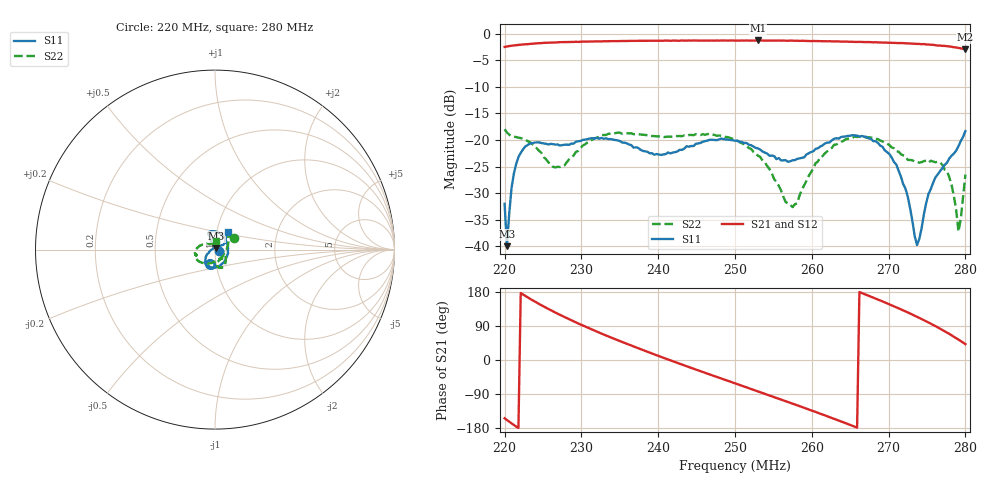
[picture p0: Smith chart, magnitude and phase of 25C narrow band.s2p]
!Agilent Technologies,E8362C,SG49020144,A.09.33.09
!Agilent E8362C: A.09.33.09
!Date: Friday, October 10, 2025 09:41:16
!Correction: S11(Full 2 Port(1,2))
!S21(Full 2 Port(1,2))
!S12(Full 2 Port(1,2))
!S22(Full 2 Port(1,2))
!S2P File: Measurements: S11, S21, S12, S22:
# Hz S  dB  R 50
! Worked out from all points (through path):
!   201 points, 220 MHz to 280 MHz, reference 50 ohm
!   highest |S21| = -1.26 dB at 253 MHz (marker M1); lowest = -2.9 dB at 280 MHz (marker M2)
!   lowest |S11| = -40.0 dB at 220.3 MHz (marker M3), VSWR 1.02, Z = 50.8 + j0.655 ohm
!   |S11| at or under -10 dB: start of sweep to end of sweep
!   |S22| runs from -37.2 to -18.0 dB; largest |S21 - S12| = 0.0071
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2.2e8  -32.01 -15.6  -2.48 -153.7  -2.50 -153.7  -17.98 32.0
2.203e8  -40.00 40.1  -2.39 -158.3  -2.40 -158.2  -18.59 36.2
2.212e8  -26.37 116.5  -2.20 -171.4  -2.19 -171.3  -19.40 44.6
2.224e8  -21.77 111.1  -2.02 172.8  -2.03 172.6  -19.82 45.1
2.266e8  -20.87 107.7  -1.64 125.3  -1.65 125.5  -25.16 -32.7
2.302e8  -19.97 111.6  -1.48 90.9  -1.48 90.8  -21.03 -118.9
2.344e8  -20.00 85.4  -1.38 54.7  -1.38 54.8  -18.72 -152.7
2.401e8  -22.73 5.7  -1.30 10.2  -1.31 10.4  -19.32 -163.6
2.446e8  -21.14 -66.2  -1.26 -23.0  -1.28 -22.8  -19.09 -164.6
2.5e8  -20.12 -111.2  -1.29 -61.6  -1.29 -61.6  -19.87 175.2
2.53e8  -21.58 -122.1  -1.26 -82.8  -1.31 -82.8  -22.98 155.9
2.575e8  -23.83 -105.0  -1.31 -115.1  -1.32 -115.2  -32.65 49.5
2.602e8  -22.13 -91.7  -1.36 -135.0  -1.36 -135.0  -25.32 -21.3
2.65e8  -19.22 -103.0  -1.51 -171.3  -1.50 -171.3  -19.67 -61.4
2.701e8  -22.64 -135.7  -1.68 146.9  -1.70 147.1  -20.95 -81.9
2.722e8  -29.18 -159.4  -1.79 128.2  -1.79 128.1  -23.10 -76.1
2.737e8  -39.78 122.1  -1.91 114.0  -1.91 114.1  -24.13 -63.1
2.752e8  -30.15 44.1  -2.03 99.0  -2.03 99.0  -24.23 -52.4
2.776e8  -24.28 33.4  -2.34 72.4  -2.35 72.7  -25.87 -49.9
2.785e8  -22.57 39.3  -2.54 61.6  -2.51 61.7  -30.55 -40.8
2.791e8  -21.18 45.9  -2.66 53.9  -2.67 54.0  -37.20 -3.9
2.8e8  -18.32 53.6  -2.93 41.8  -2.94 41.8  -26.52 80.9
